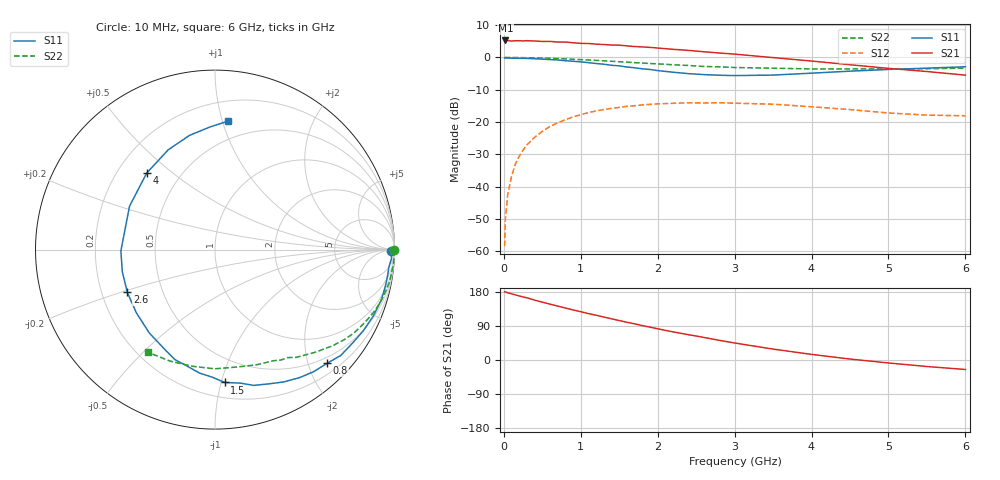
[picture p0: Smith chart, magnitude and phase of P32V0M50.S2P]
! SIEMENS Small Signal Semiconductors
! BFP181
! Si NPN RF Bipolar Junction Transistor in SOT143
! VCE = 2 V  IC = 0.5 mA
! Common Emitter S-Parameters:  March  1996
# GHz  S  MA  R  50
!  f  S11  S21  S12  S22
! GHz  MAG  ANG  MAG  ANG  MAG  ANG  MAG  ANG
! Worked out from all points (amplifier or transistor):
!   36 points, 10 MHz to 6 GHz, reference 50 ohm
!   highest |S21| = 5.3 dB at 20 MHz (marker M1)
!   |S21| within 3 dB of that: start of sweep to 2.353 GHz
!   unconditionally stable (mu >= 1): 3.697 GHz to end of sweep
!   at 250 MHz: K = 0.08, MSG = 16.9 dB, |S12| = -28.7 dB
!   at 1.4 GHz: K = 0.44, MSG = 9.8 dB, |S12| = -15.8 dB
!   at 6 GHz: K = 1.47, MAG = 2.2 dB, |S12| = -18.0 dB
!   S11 on the Smith chart (normalised r, x): 10 MHz: 81, -46; 800 MHz: 0.38, -2.34; 1.5 GHz: 0.31, -1.03; 2.6 GHz: 0.31, -0.21; 4 GHz: 0.32, +0.41; 6 GHz: 0.35, +1.04
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0.01  0.9815 -0.6  1.82 179.9  0.0012 85.2  0.9997 -0.2
0.02  0.9797 -1.2  1.834 179.6  0.0032 89.6  0.9995 -0.5
0.05  0.9855 -2.6  1.825 177.4  0.0074 90.9  0.9986 -1.4
0.1  0.9738 -5.8  1.796 174.6  0.0145 84.6  0.9981 -2.8
0.15  0.9724 -8.7  1.816 171.9  0.0224 84.0  0.9972 -4.1
0.2  0.9711 -11.5  1.816 169.0  0.0296 81.6  0.996 -5.5
0.3  0.9672 -17.2  1.819 164.2  0.0444 77.6  0.9917 -8.3
0.4  0.9561 -22.9  1.799 158.0  0.0582 73.8  0.987 -11.1
0.6  0.9267 -34.2  1.774 147.4  0.0855 65.8  0.9707 -16.4
0.8  0.8898 -45.4  1.734 137.2  0.1088 58.0  0.9505 -21.5
1.1  0.8306 -62.6  1.645 122.4  0.1403 47.0  0.9142 -28.6
1.5  0.7422 -85.8  1.551 104.2  0.1687 33.8  0.8587 -37.3
1.9  0.6524 -110.0  1.433 86.7  0.1879 22.6  0.8067 -44.6
2.2  0.5915 -128.2  1.336 74.2  0.1953 15.0  0.7712 -49.7
2.6  0.5436 -154.0  1.226 59.6  0.1977 6.3  0.7257 -56.0
3  0.5245 -179.2  1.127 44.9  0.196 -2.2  0.6988 -62.4
3.5  0.534 153.1  0.995 28.8  0.1891 -10.2  0.6821 -70.3
4  0.5716 131.7  0.881 14.8  0.1726 -16.5  0.6651 -79.7
4.5  0.6142 115.1  0.772 2.5  0.1561 -21.2  0.6642 -90.1
5  0.6519 102.6  0.678 -7.8  0.1382 -21.3  0.6621 -100.9
5.5  0.6831 92.5  0.606 -17.2  0.1282 -17.6  0.6696 -111.8
6  0.7185 84.4  0.533 -25.0  0.1253 -13.5  0.6836 -123.1
